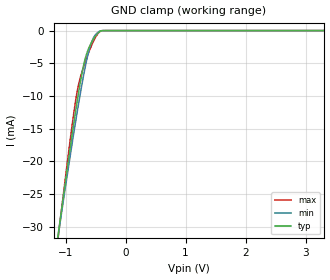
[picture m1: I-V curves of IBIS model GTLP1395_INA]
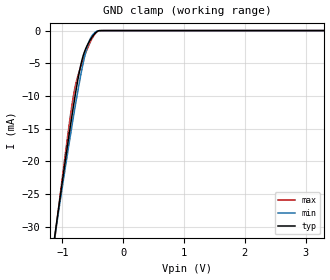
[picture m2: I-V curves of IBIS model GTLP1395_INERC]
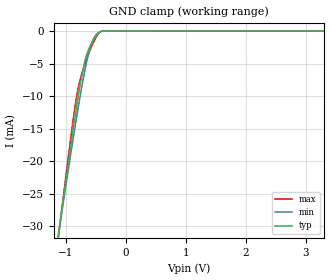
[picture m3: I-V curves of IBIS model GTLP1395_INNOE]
| TEXAS INSTRUMENTS INCORPORATED
| Standard Linear and Logic Group
| IBIS Model of SN74GTLP1395
| 2 1-BIT LVTTL-TO-GTLP ADJUSTABLE-EDGE-RATE BUS TRANSCEIVERS
| WITH SPLIT LVTTL PORT, FEEDBACK PATH, AND SELECTABLE POLATIRY
| This file contains package information for the following:
|  TVSOP 20-pin (DGV) package as [Component] GTLP1395_DGV
|  TSSOP 20-pin (PW) package as [Component] GTLP1395_PW
|  SOIC  20-pin  (DW) package as [Component] GTLP1395_DW
|  VFBGA 20-pin  (GQN) package as [Component] GTLP1395_GQN
| This device can be powered at the following Vccs:
|  3.3 volt Vcc
| This file provides unique models under the [Model Selector] for each Vcc.
| For operation at a specific Vcc, select the appropriate model after each
| [Model Selector] keyword.
[IBIS Ver]   3.2
[Comment char]  |_char
[File Name]   sn74gtlp1395.ibs
[File Rev]   1.1 | x_die
[Date]   January 24, 2002
[Source]   Data created from TI-SPICE simulations at TI-SLL.
[Notes]   The following is an IBIS list for the GTLP1395.
   Please contact sllibis@ti.com with questions and
   comments concerning SLL IBIS models.
   -As there is no power clamp diode in the Input Model,
   we removed the Pwr Clamp table data from the Input Models
[Disclaimer] Property of Texas Instruments Incorporated.  Unauthorized
   reproduction and/or distribution is strictly prohibited.
   This product is protected under copyright law.
   Created  2001, (C) Copyright  2001, Texas Instruments
   Incorporated, All Rights Reserved
   UNLESS THERE IS A SIGNED, WRITTEN AGREEMENT TO THE
   CONTRARY, TEXAS INSTRUMENTS (TI) IS PROVIDING THE IBIS
   MODELS  AND WITHOUT ANY WARRANTY, EXPRESSED OR
   IMPLIED.  TI assumes no liability for:
   1) the accuracy of the IBIS models provided to your
   company;
   2) the proper functioning of these IBIS Models in your
   design or for any resulting applications; or
   3) infringement of patents, copyrights or intellectual
   property rights resulting from your use of these IBIS
   models.
   TI provides IBIS Models as a service to our customers.
   You and your company shall not distribute, sell or give
   these models to anyone else without prior written
   permission from TI.
   TI reserves the right to make changes to our products or
   to discontinue any semiconductor product or service
   without notice, and advises our customers to obtain the
   latest version of relevant information to verify, before
   placing orders, that the information being relied on is
   current.
   Please be aware that your receipt and use of the IBIS
   information provided shall serve as acceptance of these
   terms and conditions.  If you do not accept these terms,
   you should return or destroy the IBIS models and any
   other accompanying information immediately.
| Component GTLP1395_DGV 20-pin TVSOP
[Component]   GTLP1395_DGV
[Manufacturer]   Texas Instruments, Inc.
[Package]
|   typ   min   max
R_pkg   4.400e-02   3.800e-02   4.800e-02
L_pkg   2.561e-09   2.236e-09   2.961e-09
C_pkg   3.420e-13   2.640e-13   4.460e-13
[Pin]   signal_name   model_name   R_pin   L_pin   C_pin
1   1Y   GTLP1395_OUTY   4.400e-02   2.935e-09   4.170e-13
2   1TNC   GTLP1395_INTNC   4.200e-02   2.869e-09   4.460e-13
3   2Y   GTLP1395_OUTY   4.300e-02   2.399e-09   3.160e-13
4   GND   GND   4.400e-02   2.236e-09   2.650e-13
5   1NOEAB   GTLP1395_INNOE   4.600e-02   2.278e-09   2.640e-13
6   VCC   POWER   4.500e-02   2.274e-09   2.640e-13
7   1A   GTLP1395_INA   4.400e-02   2.285e-09   2.690e-13
8   GND   GND   4.300e-02   2.452e-09   3.200e-13
9   2A   GTLP1395_INA   4.400e-02   2.900e-09   4.460e-13
10   2NOEAB   GTLP1395_INNOE   4.400e-02   2.961e-09   4.180e-13
11   BIASVCC   GTLP1395_INBV   4.500e-02   2.954e-09   4.180e-13
12   VREF   GTLP1395_INVREF   4.200e-02   2.847e-09   4.430e-13
13   GND   GND   4.500e-02   2.453e-09   3.190e-13
14   2B   GTLP1395_IOB   4.500e-02   2.297e-09   2.690e-13
15   ERC   GTLP1395_INERC   4.800e-02   2.334e-09   2.680e-13
16   1B   GTLP1395_IOB   4.800e-02   2.335e-09   2.670e-13
17   GND   GND   4.600e-02   2.299e-09   2.680e-13
18   2NOEBY   GTLP1395_INNOE   4.600e-02   2.457e-09   3.200e-13
19   2TNC   GTLP1395_INTNC   4.300e-02   2.848e-09   4.410e-13
20   1NOEBY   GTLP1395_INNOE   3.800e-02   2.812e-09   4.080e-13
|   Component   GTLP1395_GQN   20-pin   VFBGA
[Component]   GTLP1395_GQN
[Manufacturer]   Texas   Instruments,   Inc.
[Package]
|   typ   min   max
R_pkg   4.3000E-02   3.3000E-02   6.1000E-02
L_pkg   1.3170E-09   8.9600E-10   2.0880E-09
C_pkg   1.1300E-13   6.4000E-14   1.9000E-13
[Pin]   signal_name   model_name   R_pin   L_pin   C_pin
1   1Y   GTLP1395_OUTY   3.8000E-02   1.1990E-09   1.2100E-13
2   1TNC   GTLP1395_INTNC  4.0000E-02   1.0670E-09   1.0200E-13
3   2Y   GTLP1395_OUTY   6.1000E-02   1.9990E-09   1.9000E-13
4   GND   GND   3.3000E-02   9.6300E-10   7.1000E-14
5   1NOEAB   GTLP1395_INNOE  4.9000E-02   1.5230E-09   1.2300E-13
6   VCC   POWER   3.3000E-02   8.9600E-10   6.4000E-14
7   1A   GTLP1395_INA   6.1000E-02   1.8990E-09   1.6400E-13
8   GND   GND   3.3000E-02   8.9800E-10   6.7000E-14
9   2A   GTLP1395_INA   4.9000E-02   1.5140E-09   1.2800E-13
10   2NOEAB   GTLP1395_INNOE  3.6000E-02   1.0060E-09   9.4000E-14
11   BIASVCC  GTLP1395_INBV   4.9000E-02   1.6830E-09   1.4600E-13
12   VREF   GTLP1395_INVREF 3.3000E-02   1.1210E-09   8.9000E-14
13   GND   GND   6.1000E-02   2.0880E-09   1.7300E-13
14   2B   GTLP1395_IOB   3.3000E-02   1.0270E-09   7.1000E-14
15   ERC   GTLP1395_INERC  4.9000E-02   1.5580E-09   1.2400E-13
16   1B   GTLP1395_IOB   3.3000E-02   9.2800E-10   6.7000E-14
17   GND   GND   6.1000E-02   1.9210E-09   1.7700E-13
18   2NOEBY   GTLP1395_INNOE  3.3000E-02   9.0100E-10   7.7000E-14
19   2TNC   GTLP1395_INTNC  3.7000E-02   9.9000E-10   9.8000E-14
20   1NOEBY   GTLP1395_INNOE  3.5000E-02   1.1680E-09   1.1900E-13
| Component GTLP1395_PW 20-pin TSSOP
[Component]   GTLP1395_PW
[Manufacturer]   Texas Instruments, Inc.
[Package]
|   typ   min   max
R_pkg   4.500e-02   3.600e-02   5.700e-02
L_pkg   2.694e-09   2.290e-09   3.177e-09
C_pkg   1.560e-13   7.600e-14   2.590e-13
[Pin]   signal_name   model_name   R_pin   L_pin   C_pin
1   1Y   GTLP1395_OUTY   3.600e-02   3.045e-09   2.590e-13
2   1TNC   GTLP1395_INTNC   5.100e-02   3.013e-09   1.890e-13
3   2Y   GTLP1395_OUTY   4.400e-02   2.695e-09   1.640e-13
4   GND   GND   4.700e-02   2.362e-09   7.900e-14
5   1NOEAB   GTLP1395_INNOE   4.700e-02   2.333e-09   8.600e-14
6   VCC   POWER   4.700e-02   2.298e-09   8.500e-14
7   1A   GTLP1395_INA   4.700e-02   2.351e-09   7.900e-14
8   GND   GND   4.400e-02   2.706e-09   1.650e-13
9   2A   GTLP1395_INA   4.900e-02   2.999e-09   1.880e-13
10   2NOEAB   GTLP1395_INNOE   3.900e-02   3.039e-09   2.570e-13
11   BIASVCC   GTLP1395_INBV   3.800e-02   3.044e-09   2.580e-13
12   VREF   GTLP1395_INVREF   5.700e-02   3.177e-09   1.990e-13
13   GND   GND   4.400e-02   2.825e-09   1.730e-13
14   2B   GTLP1395_IOB   4.700e-02   2.429e-09   8.300e-14
15   ERC   GTLP1395_INERC   4.900e-02   2.383e-09   9.000e-14
16   1B   GTLP1395_IOB   4.900e-02   2.347e-09   8.900e-14
17   GND   GND   4.700e-02   2.290e-09   7.600e-14
18   2NOEBY   GTLP1395_INNOE   4.500e-02   2.613e-09   1.580e-13
19   2TNC   GTLP1395_INTNC   4.400e-02   2.883e-09   1.810e-13
20   1NOEBY   GTLP1395_INNOE   3.900e-02   3.044e-09   2.560e-13
| Component GTLP1395_DW 20-pin SOIC
[Component]   GTLP1395_DW
[Manufacturer]   Texas Instruments, Inc.
[Package]
|   typ   min   max
R_pkg   3.800e-02   3.300e-02   4.500e-02
L_pkg   5.012e-09   4.110e-09   6.349e-09
C_pkg   7.170e-13   5.300e-13   8.680e-13
[Pin]   signal_name   model_name   R_pin   L_pin   C_pin
1   1Y   GTLP1395_OUTY   4.200e-02   6.336e-09   8.650e-13
2   1TNC   GTLP1395_INTNC   4.300e-02   5.542e-09   8.670e-13
3   2Y   GTLP1395_OUTY   3.400e-02   4.714e-09   7.320e-13
4   GND   GND   3.400e-02   4.377e-09   5.910e-13
5   1NOEAB   GTLP1395_INNOE   3.600e-02   4.130e-09   5.330e-13
6   VCC   POWER   3.500e-02   4.111e-09   5.300e-13
7   1A   GTLP1395_INA   3.400e-02   4.284e-09   5.830e-13
8   GND   GND   3.400e-02   4.634e-09   7.260e-13
9   2A   GTLP1395_INA   4.000e-02   5.518e-09   8.650e-13
10   2NOEAB   GTLP1395_INNOE   4.300e-02   6.349e-09   8.660e-13
11   BIASVCC   GTLP1395_INBV   4.100e-02   6.281e-09   8.610e-13
12   VREF   GTLP1395_INVREF   4.500e-02   5.561e-09   8.680e-13
13   GND   GND   3.300e-02   4.778e-09   7.420e-13
14   2B   GTLP1395_IOB   3.500e-02   4.414e-09   5.960e-13
15   ERC   GTLP1395_INERC   3.500e-02   4.110e-09   5.330e-13
16   1B   GTLP1395_IOB   3.600e-02   4.130e-09   5.330e-13
17   GND   GND   3.400e-02   4.377e-09   5.910e-13
18   2NOEBY   GTLP1395_INNOE   3.400e-02   4.714e-09   7.310e-13
19   2TNC   GTLP1395_INTNC   4.300e-02   5.569e-09   8.680e-13
20   1NOEBY   GTLP1395_INNOE   4.200e-02   6.308e-09   8.640e-13
| NOTE:  The [Diff Pin] section is commented out because the ibischk3 program
|   currently flags it as an Error when it shouldn't
| [Diff Pin]  inv_pin   vdiff   tdelay_typ
|16   12   100mV   NA
|14   12   100mV   NA
| Model GTLP1395_IOB
[Model Selector]   GTLP1395_IOB
GTLP1395_IOB_SLOW   3.3 volt Vcc  Slow ERC
GTLP1395_IOB_FAST   3.3 volt Vcc  Fast ERC
| Models and submodels in the file (9): GTLP1395_INA (Input), GTLP1395_INERC (Input), GTLP1395_INNOE (Input), GTLP1395_INVREF (Input), GTLP1395_INTNC (Input), GTLP1395_INBV (Input), GTLP1395_IOB_SLOW (I/O_open_drain), GTLP1395_IOB_FAST (I/O_open_drain), GTLP1395_OUTY (3-state)
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[Model]   GTLP1395_INA
Model_type  Input
Vinl = 0.8
Vinh = 2.0
| variable   typ   min   max
C_comp   2.48pF   1.81pF   3.65pF
[Temperature Range]   40   100   -40
| Ambient temperature   25   85   -40
[Voltage range]   3.3   3.15   3.45
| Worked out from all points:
|   GND clamp passes 1 mA (typ) near -0.51 V on its own axis
[GND Clamp]
| GTLP1395_INA
|   Voltage   I(typ)   I(min)   I(max)
-5.5V     -354.3mA   -327.1mA   -395.8mA
-1.15V    -33.04mA   -33.05mA   -33.71mA
-1.11V    -30.33mA   -30.56mA   -30.64mA
-890mV    -15.89mA   -17.25mA   -14.45mA
-835mV    -12.51mA   -14.09mA   -10.9mA
-795mV    -10.17mA   -11.85mA   -8.783mA
-695mV    -5.144mA   -6.648mA   -5.431mA
-610mV    -2.623mA   -3.059mA   -3.251mA
-545mV    -1.467mA   -1.304mA   -1.835mA
-460mV    -389.9uA   -251.6uA   -457.8uA
-365mV    -3.918uA   -10.79uA   -4.011uA
3.3V      166.6pA    582.9pA    1.325nA
[Model]   GTLP1395_INERC
Model_type  Input
Vinl = 0.8
Vinh = 2.0
| variable   typ   min   max
C_comp   2.25pF   1.68pF   3.40pF
[Temperature Range]   40   100   -40
| Ambient temperature   25   85   -40
[Voltage range]   3.3   3.15   3.45
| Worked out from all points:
|   GND clamp passes 1 mA (typ) near -0.51 V on its own axis
[GND Clamp]
| GTLP1395_INERC
|   Voltage   I(typ)   I(min)   I(max)
-5.5V     -354.3mA   -327.1mA   -395.8mA
-1.15V    -33.04mA   -33.05mA   -33.71mA
-1.11V    -30.33mA   -30.56mA   -30.64mA
-890mV    -15.89mA   -17.25mA   -14.45mA
-835mV    -12.51mA   -14.09mA   -10.9mA
-795mV    -10.17mA   -11.85mA   -8.783mA
-695mV    -5.144mA   -6.648mA   -5.431mA
-610mV    -2.623mA   -3.059mA   -3.251mA
-545mV    -1.467mA   -1.304mA   -1.835mA
-460mV    -389.9uA   -251.6uA   -457.8uA
-365mV    -3.918uA   -10.79uA   -4.011uA
3.3V      166.6pA    582.9pA    1.325nA
[Model]   GTLP1395_INNOE
Model_type  Input
Vinl = 0.8
Vinh = 2.0
| variable   typ   min   max
C_comp   2.85pF   1.91pF   4.05pF
[Temperature Range]   40   100   -40
| Ambient temperature   25   85   -40
[Voltage range]   3.3   3.15   3.45
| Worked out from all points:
|   GND clamp passes 1 mA (typ) near -0.51 V on its own axis
[GND Clamp]
| GTLP1395_INNOE
|   Voltage   I(typ)   I(min)   I(max)
-5.5V     -354.3mA   -327.1mA   -395.8mA
-1.15V    -33.04mA   -33.05mA   -33.71mA
-1.11V    -30.33mA   -30.56mA   -30.64mA
-890mV    -15.89mA   -17.25mA   -14.45mA
-835mV    -12.51mA   -14.09mA   -10.9mA
-795mV    -10.17mA   -11.85mA   -8.783mA
-695mV    -5.144mA   -6.648mA   -5.431mA
-610mV    -2.623mA   -3.059mA   -3.251mA
-545mV    -1.467mA   -1.304mA   -1.835mA
-460mV    -389.9uA   -251.6uA   -457.8uA
-365mV    -3.918uA   -10.79uA   -4.011uA
3.3V      166.6pA    582.9pA    1.325nA
